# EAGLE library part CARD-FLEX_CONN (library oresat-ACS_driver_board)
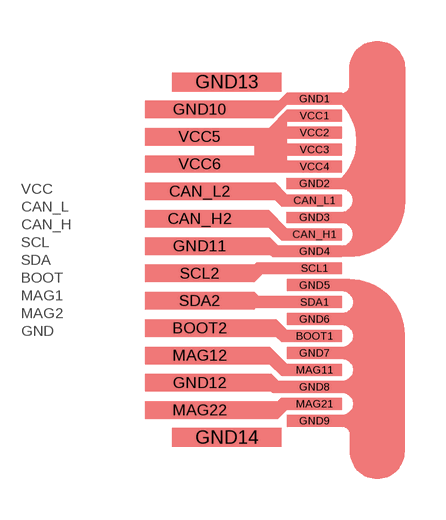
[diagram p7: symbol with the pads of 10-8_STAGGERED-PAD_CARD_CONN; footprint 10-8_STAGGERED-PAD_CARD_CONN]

Designator prefix -

## CARD-FLEX_CONNCARD-FLEX_CONN  [10-8_STAGGERED-PAD_CARD_CONN]
BOOT1  BOOT
BOOT2  BOOT
CAN_H1  CAN_H
CAN_H2  CAN_H
CAN_L1  CAN_L
CAN_L2  CAN_L
GND1  GND
GND2  GND
GND3  GND
GND4  GND
GND5  GND
GND6  GND
GND7  GND
GND8  GND
GND9  GND
GND10  GND
GND11  GND
GND12  GND
GND13  GND
GND14  GND
MAG11  MAG1
MAG12  MAG1
MAG21  MAG2
MAG22  MAG2
SCL1  SCL
SCL2  SCL
SDA1  SDA
SDA2  SDA
VCC1  VCC
VCC2  VCC
VCC3  VCC
VCC4  VCC
VCC5  VCC
VCC6  VCC

## Footprint 10-8_STAGGERED-PAD_CARD_CONN (pad centres in mm)
smd 2 x 0.4: BOOT1 0.7,-2.79; CAN_H1 0.7,0.93; CAN_L1 0.7,2.17; GND1 0.7,5.89; GND2 0.7,2.79; GND3 0.7,1.55; GND4 0.7,0.31; GND5 0.7,-0.93; GND6 0.7,-2.17; GND7 0.7,-3.41; GND8 0.7,-4.65; GND9 0.7,-5.89; MAG11 0.7,-4.03; MAG21 0.7,-5.27; SCL1 0.7,-0.31; SDA1 0.7,-1.55; VCC1 0.7,5.27; VCC2 0.7,4.65; VCC3 0.7,4.03; VCC4 0.7,3.41
smd 4 x 0.6: BOOT2 -3.5,-2.5; CAN_H2 -3.5,1.5; CAN_L2 -3.5,2.5; GND10 -3.5,5.5; GND11 -3.5,0.5; GND12 -3.5,-4.5; MAG12 -3.5,-3.5; MAG22 -3.5,-5.5; SCL2 -3.5,-0.5; SDA2 -3.5,-1.5; VCC5 -3.5,4.5; VCC6 -3.5,3.5
smd 4 x 0.7: GND13 -2.5,6.5; GND14 -2.5,-6.5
